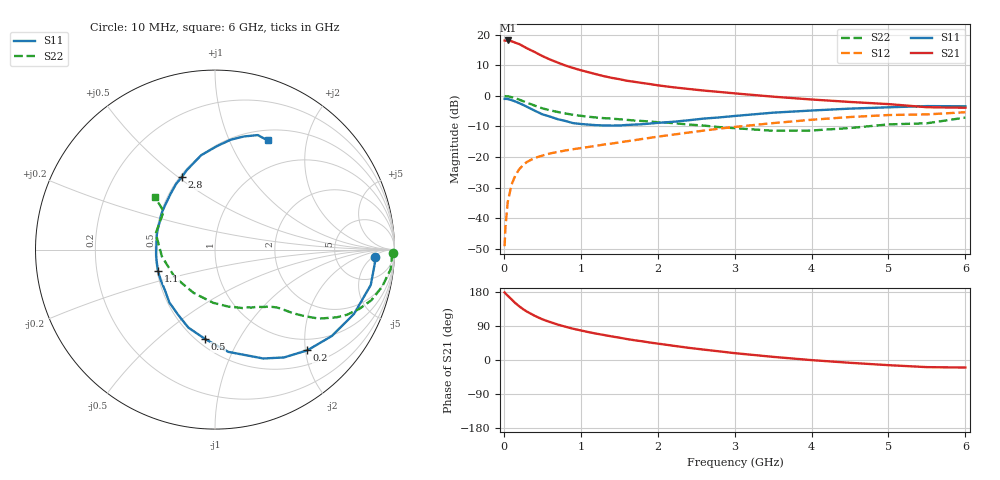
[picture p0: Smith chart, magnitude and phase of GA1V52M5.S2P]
! Infineon Technologies  Discrete & RF Semiconductors
! BF775
! Si NPN RF Bipolar Junction Transistor in SOT23
! VCE = 1.5 V  IC = 2.5 mA
! Common Emitter S-Parameters:  May  1996
# GHz  S  MA  R  50
!  f  S11  S21  S12  S22
! GHz  MAG  ANG  MAG  ANG  MAG  ANG  MAG  ANG
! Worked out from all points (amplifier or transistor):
!   36 points, 10 MHz to 6 GHz, reference 50 ohm
!   highest |S21| = 18.1 dB at 50 MHz (marker M1)
!   |S21| within 3 dB of that: start of sweep to 336.6 MHz
!   unconditionally stable (mu >= 1): 1.012 GHz to end of sweep
!   at 250 MHz: K = 0.33, MSG = 19.4 dB, |S12| = -22.6 dB
!   at 1.4 GHz: K = 1.15, MAG = 8.4 dB, |S12| = -15.6 dB
!   at 6 GHz: K = 1.03, MAG = -0.3 dB, |S12| = -5.3 dB
!   S11 on the Smith chart (normalised r, x): 10 MHz: 15, -6; 200 MHz: 0.76, -2.04; 500 MHz: 0.55, -0.73; 1.1 GHz: 0.51, -0.14; 2.8 GHz: 0.51, +0.52; 6 GHz: 0.63, +1.40
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0.01  0.8933 -2.5  8.025 178.3  0.0035 88.2  0.9942 -1.2
0.02  0.8936 -5.0  7.944 175.8  0.007 87.5  0.9863 -2.5
0.05  0.89 -12.8  8.051 169.8  0.0182 83.6  0.9847 -6.4
0.1  0.8535 -24.8  7.82 160.1  0.0354 76.4  0.9538 -12.5
0.15  0.8095 -36.5  7.391 150.1  0.0503 69.5  0.9161 -17.9
0.2  0.7613 -47.5  7.024 141.8  0.0633 64.6  0.8688 -22.4
0.25  0.7133 -57.4  6.495 134.2  0.074 59.5  0.8196 -26.3
0.3  0.6636 -66.1  5.999 127.7  0.0833 56.4  0.7758 -29.1
0.4  0.5745 -82.6  5.217 116.8  0.0965 50.9  0.6949 -33.6
0.5  0.5004 -96.5  4.482 107.4  0.1057 47.8  0.6264 -36.4
0.6  0.4591 -108.9  3.932 100.2  0.1146 45.5  0.5808 -38.3
0.7  0.4164 -119.8  3.505 93.5  0.1215 44.4  0.5462 -39.7
0.9  0.3593 -140.9  2.859 82.5  0.1344 43.8  0.4911 -41.9
1.1  0.3393 -159.3  2.436 73.7  0.1463 44.2  0.4566 -44.5
1.3  0.3294 -174.2  2.102 66.0  0.1601 44.4  0.4329 -47.1
1.6  0.335 165.2  1.768 55.3  0.1815 44.8  0.4058 -51.9
2.2  0.3772 135.9  1.383 37.7  0.2326 44.2  0.3595 -64.9
2.8  0.4447 114.5  1.16 22.8  0.2913 40.6  0.3088 -83.8
3.5  0.5317 98.3  0.971 8.3  0.3591 33.5  0.2689 -116.4
4.5  0.6194 81.7  0.796 -7.4  0.4512 20.9  0.2984 -172.7
5.5  0.6812 69.5  0.653 -18.8  0.4982 6.1  0.3568 143.3
6  0.6752 64.2  0.64 -19.9  0.5406 2.1  0.4422 138.9
